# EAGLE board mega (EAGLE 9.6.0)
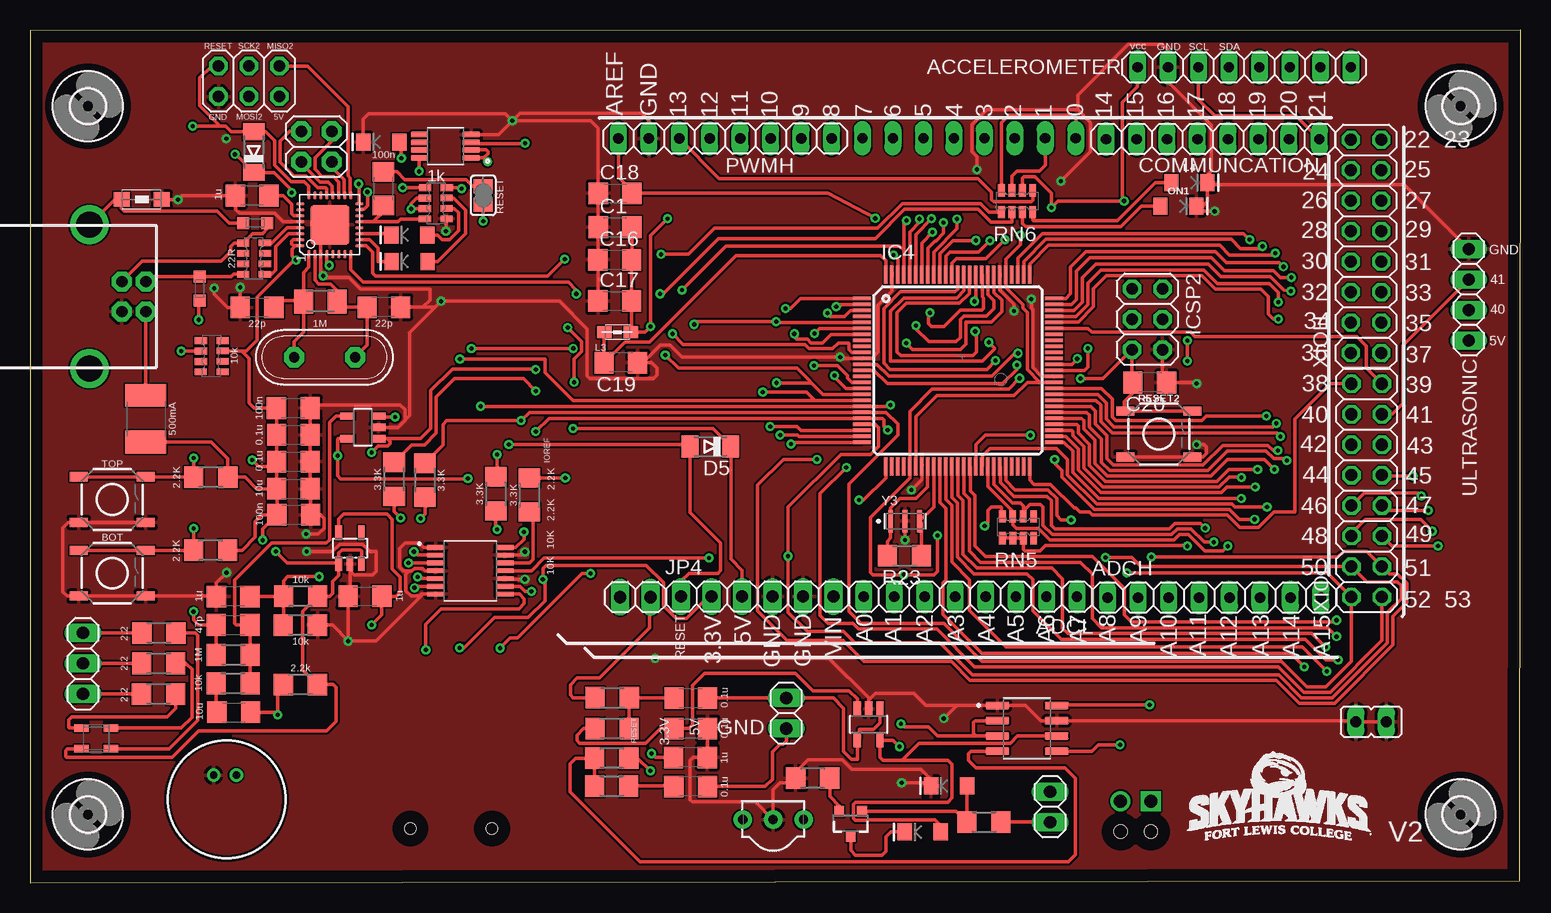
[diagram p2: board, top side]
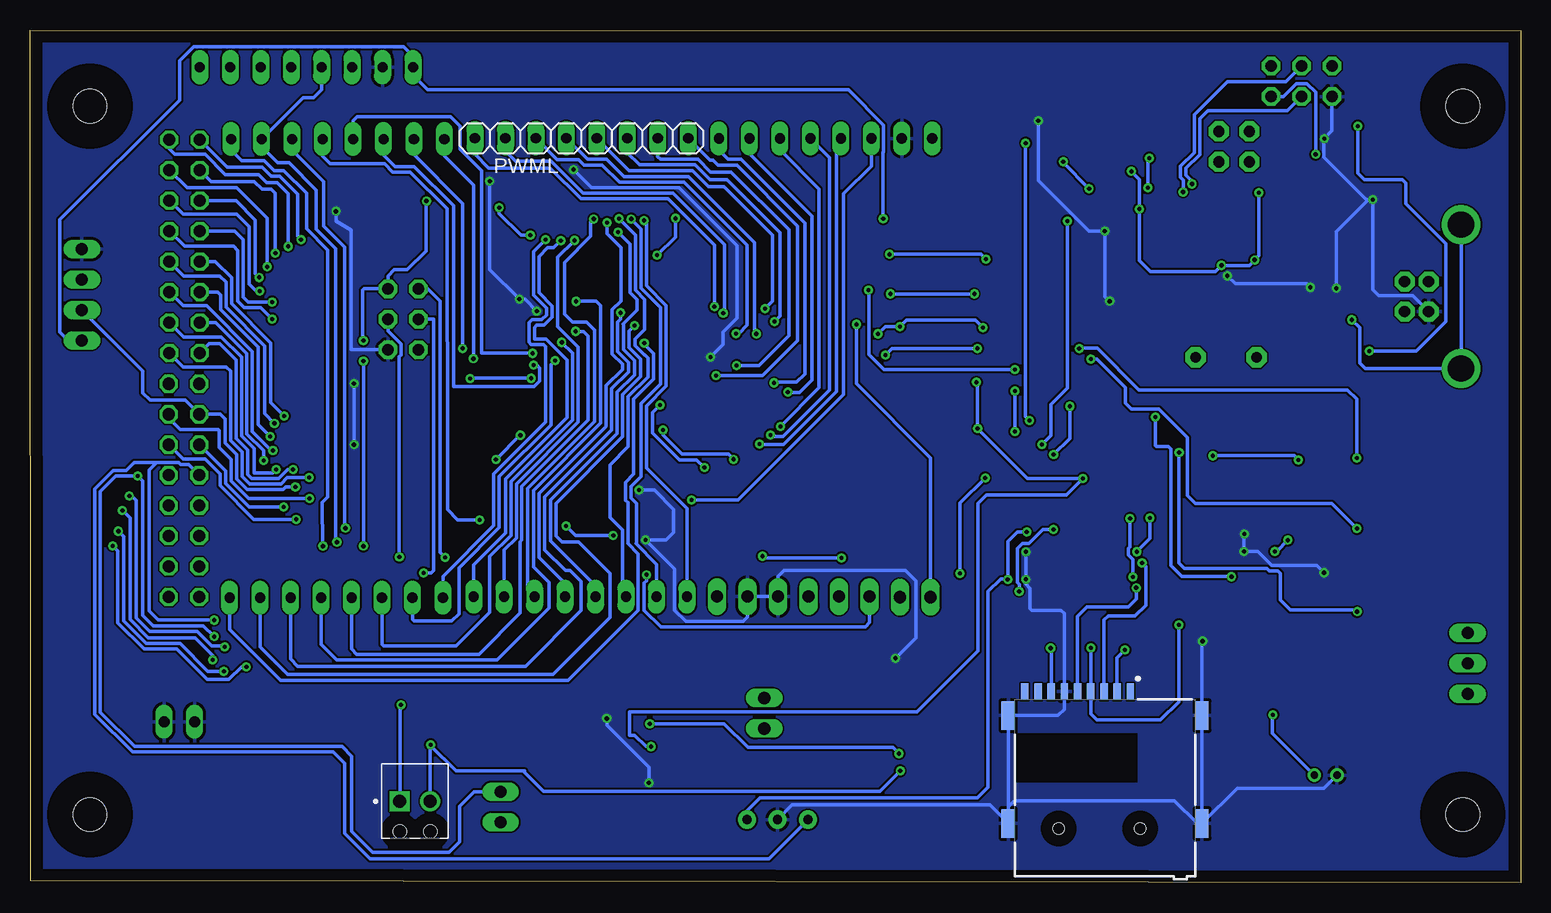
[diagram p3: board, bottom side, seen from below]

Size 124.26 x 71.1 mm. Coordinates in mm from the lower left corner, seen from the top.
Outline: 0,0 124.19,0.17 124.26,71.1 0.01,71.05 0,0
Copper layers (1*16): Top 0.035mm / dielectric 1.5mm / Bottom 0.035mm
Design rules "default": minimum track width 6mil, minimum drill 0.35mm, track to track 6mil, track to pad 6mil, pad to pad 6mil, via to via 6mil, smd to smd 6mil, copper to edge 40mil, drill to drill 6mil, minimum pad ring 10mil, minimum via ring 8mil, stop-mask expansion 4mil, vias tented up to drill 0mil, thermal gap 10mil
Net classes: 0 default: width 0.305 mm

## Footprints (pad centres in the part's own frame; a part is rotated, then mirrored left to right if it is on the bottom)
SMARTPRJ_1X08 = drill 0.85 pad 1.422 long: 1 -8.89,0; 2 -6.35,0; 3 -3.81,0; 4 -1.27,0; 5 1.27,0; 6 3.81,0; 7 6.35,0; 8 8.89,0
TACTILE_SWITCH_SMD_5.2MM = smd 1.524 x 0.762: 1 -2.794,1.905; 2 2.794,1.905; 3 -2.794,-1.905; 4 2.794,-1.905
SMARTPRJ_C1206 = smd 1.6 x 1.8: 1 -1.4,0; 2 1.4,0
LED-1206 = smd 1.2 x 1.4: A -1.5,0; C 1.5,0
DIODE_MINIMELF = smd 1.4 x 1.8: A 1.7,0; C -1.7,0
RCL_L1812 = smd 1.9 x 3.4: 1 -1.95,0; 2 1.95,0
2,8 = hole 2.8: 0,0
SOT23-5 = smd 0.6 x 1.2: 1 -0.95,-1.306; 2 0,-1.306; 3 0.95,-1.306; 4 0.95,1.306; 5 -0.95,1.306
INTEGRATEDCIRCUITS_TQFP100 = smd 1.5 x 0.3: 1 -8,6; 2 -8,5.5; 3 -8,5; 4 -8,4.5; 5 -8,4; 6 -8,3.5; 7 -8,3; 8 -8,2.5; 9 -8,2; 10 -8,1.5; 11 -8,1; 12 -8,0.5; 13 -8,0; 14 -8,-0.5; 15 -8,-1; 16 -8,-1.5; 17 -8,-2; 18 -8,-2.5; 19 -8,-3; 20 -8,-3.5; 21 -8,-4; 22 -8,-4.5; 23 -8,-5; 24 -8,-5.5; 25 -8,-6; 51 8,-6; 52 8,-5.5; 53 8,-5; 54 8,-4.5; 55 8,-4; 56 8,-3.5; 57 8,-3; 58 8,-2.5; 59 8,-2; 60 8,-1.5; 61 8,-1; 62 8,-0.5; 63 8,0; 64 8,0.5; 65 8,1; 66 8,1.5; 67 8,2; 68 8,2.5; 69 8,3; 70 8,3.5; 71 8,4; 72 8,4.5; 73 8,5; 74 8,5.5; 75 8,6 | smd 0.3 x 1.5: 26 -6,-8; 27 -5.5,-8; 28 -5,-8; 29 -4.5,-8; 30 -4,-8; 31 -3.5,-8; 32 -3,-8; 33 -2.5,-8; 34 -2,-8; 35 -1.5,-8; 36 -1,-8; 37 -0.5,-8; 38 0,-8; 39 0.5,-8; 40 1,-8; 41 1.5,-8; 42 2,-8; 43 2.5,-8; 44 3,-8; 45 3.5,-8; 46 4,-8; 47 4.5,-8; 48 5,-8; 49 5.5,-8; 50 6,-8; 76 6,8; 77 5.5,8; 78 5,8; 79 4.5,8; 80 4,8; 81 3.5,8; 82 3,8; 83 2.5,8; 84 2,8; 85 1.5,8; 86 1,8; 87 0.5,8; 88 0,8; 89 -0.5,8; 90 -1,8; 91 -1.5,8; 92 -2,8; 93 -2.5,8; 94 -3,8; 95 -3.5,8; 96 -4,8; 97 -4.5,8; 98 -5,8; 99 -5.5,8; 100 -6,8
2X03 = drill 0.95 pad 1.55 octagon: 1 -2.54,-1.27; 2 -2.54,1.27; 3 0,-1.27; 4 0,1.27; 5 2.54,-1.27; 6 2.54,1.27
SMARTPRJ_2X03 = drill 0.95 pad 1.55 octagon: 1 -2.54,-1.27; 2 -2.54,1.27; 3 0,-1.27; 4 0,1.27; 5 2.54,-1.27; 6 2.54,1.27
GCT_MEM2075-00-140-01-A = smd 0.62 x 1.4: P1 2.58,11.42; P2 1.48,11.42; P3 0.38,11.42; P4 -0.72,11.42; P5 -1.82,11.42; P6 -2.92,11.42; P7 -4.02,11.42; P8 -5.12,11.42; P9 -6.22,11.42 | smd 1.1 x 2.4: SH1 -7.6,0.42; SH2 -7.6,9.42; SH3 8.55,9.42; SH4 8.55,0.42 | hole 0.95: -3.4,0; 3.4,0
PHOENIX_1725656 = drill 1.1 square: 1 1.5,3.1 | drill 1.1: 2 4.04,3.1 | hole 1.1: 1.5,0.56; 4.04,0.56
SMARTPRJ_2X02 = drill 0.95 pad 1.676 octagon: 1 -1.27,-1.27; 2 -1.27,1.27; 3 1.27,-1.27; 4 1.27,1.27
1X03 = drill 1.016 long: 1 -2.54,0; 2 0,0; 3 2.54,0
1X06 = drill 1.016 long: 1 -6.35,0; 2 -3.81,0; 3 -1.27,0; 4 1.27,0; 5 3.81,0; 6 6.35,0
1X02 = drill 1.016 long: 1 -1.27,0; 2 1.27,0
JP1 = drill 0.914 long: 1 0,-1.27; 2 0,1.27
WUERTH-ELEKTRONIK_1206 = smd 1.35 x 1.2: 1 -1.7,0; 2 1.65,0
INDUTTANZE_0805 = smd 1.2 x 1: 1 -1.1,0; 2 1.1,0
SOT23-3 = smd 0.8 x 0.9: 1 -0.95,-1; 2 0.95,-1; 3 0,1.1
SMARTPRJ_M1206 = smd 1.6 x 2: 1 -1.4,0; 2 1.4,0
R1206 = smd 1.6 x 1.803: 1 -1.422,0; 2 1.422,0
SMARTPRJ_R1206 = smd 1.6 x 1.803: 1 -1.422,0; 2 1.422,0
JUMPER_SJ = smd 1.168 x 1.6: 1 -0.762,0; 2 0.762,0
RESISTOR-DIL_CAY16 = smd 0.559 x 1.016: 1 -1.283,-0.934; 2 -0.408,-0.94; 3 0.462,-0.943; 4 1.322,-0.942; 5 1.318,0.874; 6 0.452,0.877; 7 -0.42,0.877; 8 -1.289,0.883
TSOP382 = drill 0.762 pad 1.524: 1 -2.54,0; 2 0,0; 3 2.54,0
SMARTPRJ_SOT23-DBV = smd 0.55 x 1.2: 1 -0.95,-1.3; 2 0,-1.3; 3 0.95,-1.3; 4 0.95,1.3; 5 -0.95,1.3
SOP65P640X120-14N = smd 1.57 x 0.41: 1 -2.87,1.95; 2 -2.87,1.3; 3 -2.87,0.65; 4 -2.87,0; 5 -2.87,-0.65; 6 -2.87,-1.3; 7 -2.87,-1.95; 8 2.87,-1.95; 9 2.87,-1.3; 10 2.87,-0.65; 11 2.87,0; 12 2.87,0.65; 13 2.87,1.3; 14 2.87,1.95
SOP65P490X110-8N = smd 1.47 x 0.48: 1 -2.15,0.975; 2 -2.15,0.325; 3 -2.15,-0.325; 4 -2.15,-0.975; 5 2.15,-0.975; 6 2.15,-0.325; 7 2.15,0.325; 8 2.15,0.975
SMARTPRJ_MLF32 = smd 0.7 x 0.28: 1 -2.45,1.75; 2 -2.45,1.25; 3 -2.45,0.75; 4 -2.45,0.25; 5 -2.45,-0.25; 6 -2.45,-0.75; 7 -2.45,-1.25; 8 -2.45,-1.75; 17 2.45,-1.75; 18 2.45,-1.25; 19 2.45,-0.75; 20 2.45,-0.25; 21 2.45,0.25; 22 2.45,0.75; 23 2.45,1.25; 24 2.45,1.75 | smd 0.28 x 0.7: 9 -1.75,-2.45; 10 -1.25,-2.45; 11 -0.75,-2.45; 12 -0.25,-2.45; 13 0.25,-2.45; 14 0.75,-2.45; 15 1.25,-2.45; 16 1.75,-2.45; 25 1.75,2.45; 26 1.25,2.45; 27 0.75,2.45; 28 0.25,2.45; 29 -0.25,2.45; 30 -0.75,2.45; 31 -1.25,2.45; 32 -1.75,2.45 | smd 3.254 x 3.254: 33 0,0
WM-62PC/62PK = drill 0.6 pad 1: 1 -2.016,0.823; 2 -2.016,-1.077
GM1WA55311A = smd 1.2 x 0.65: 1 -1.535,0.856; 2 -1.535,-0.856; 3 0.9,-0.856; 4 0.9,0.856
MYSOIC8 = smd 1.97 x 0.6: 1 -2.47,1.905; 2 -2.47,0.635; 3 -2.47,-0.635; 4 -2.47,-1.905; 5 2.47,-1.905; 6 2.47,-0.635; 7 2.47,0.635; 8 2.47,1.905
1X04 = drill 1.016 long: 1 -3.81,0; 2 -1.27,0; 3 1.27,0; 4 3.81,0
SMARTPRJ_PN61729 = drill 0.95 pad 1.676 octagon: 1 1.25,4.71; 2 -1.25,4.71; 3 -1.25,2.71; 4 1.25,2.71 | drill 2.2: P$1 -6,0; P$2 6,0
2X08 = drill 1.016 octagon: 1 -8.89,-1.27; 2 -8.89,1.27; 3 -6.35,-1.27; 4 -6.35,1.27; 5 -3.81,-1.27; 6 -3.81,1.27; 7 -1.27,-1.27; 8 -1.27,1.27; 9 1.27,-1.27; 10 1.27,1.27; 11 3.81,-1.27; 12 3.81,1.27; 13 6.35,-1.27; 14 6.35,1.27; 15 8.89,-1.27; 16 8.89,1.27
SMARTPRJ_QS = drill 0.85 pad 1.676 octagon: 1 -2.54,0; 2 2.54,0
OSC_CSTNE16M0V530000R0 = smd 0.4 x 1.9: 1 -1.2,0; 2 0,0; 3 1.2,0
VARISTOR_CT/CN0603 = smd 1 x 1: 1 -1,0; 2 1,0

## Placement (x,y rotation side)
ACCELEROMETER  8x1  [SMARTPRJ_1X08]  101.22,68 180 top
ADCH  8x1  [SMARTPRJ_1X08]  98.73,23.78 0 top
ADCL  8x1  [SMARTPRJ_1X08]  78.39,23.85 180 top
BOT  MOMENTARY-SWITCH-SPST-SMD-5.2-REDUNDANT  [TACTILE_SWITCH_SMD_5.2MM]  6.85,25.81 0 top
C1  100n  [SMARTPRJ_C1206]  48.77,54.66 0 top
C2  100n  [SMARTPRJ_C1206]  21.98,30.67 180 top
C3  1u  [SMARTPRJ_C1206]  27.93,23.9 0 top
C5  100n  [SMARTPRJ_C1206]  29.46,57.88 90 top
C7  100n  [SMARTPRJ_C1206]  21.95,39.59 0 top
C8  1u  [SMARTPRJ_C1206]  18.52,57.29 180 top
C9  22p  [SMARTPRJ_C1206]  18.93,47.98 0 top
C11  22p  [SMARTPRJ_C1206]  29.49,47.99 180 top
C12  1u  [SMARTPRJ_C1206]  16.94,23.87 180 top
C13  47p  [SMARTPRJ_C1206]  16.93,21.5 0 top
C14  1u  [SMARTPRJ_C1206]  55.06,10.45 180 top
C15  0.1u  [SMARTPRJ_C1206]  55.07,8.03 180 top
C16  100n  [SMARTPRJ_C1206]  48.74,51.95 0 top
C17  100n  [SMARTPRJ_C1206]  48.74,48.52 0 top
C18  100n  [SMARTPRJ_C1206]  48.77,57.48 0 top
C19  100n  [SMARTPRJ_C1206]  49.25,43.36 180 top
C20  22p  [SMARTPRJ_C1206]  93.34,41.71 180 top
CC1  10u  [SMARTPRJ_C1206]  21.96,32.85 0 top
CC2  10u  [SMARTPRJ_C1206]  16.98,14.22 0 top
CC3  0.1u  [SMARTPRJ_C1206]  21.95,37.35 0 top
CC4  0.1u  [SMARTPRJ_C1206]  21.95,35.11 0 top
CC5  0.1u  [SMARTPRJ_C1206]  55.08,12.86 0 top
CC6  0.1u  [SMARTPRJ_C1206]  55.08,15.41 0 top
COMMUNCATION  8x1  [SMARTPRJ_1X08]  98.6,62 0 top
D1  INFRARED  [LED-1206]  74.41,4.24 180 top
D3  CD1206-S01575  [DIODE_MINIMELF]  18.65,60.93 90 top
D4  RED  [LED-1206]  76.61,8.08 180 top
D5  CD1206-S01575  [DIODE_MINIMELF]  56.72,36.38 180 top
F1  MF-MSMF050-2 500mA  [RCL_L1812]  9.65,38.7 270 top
H1  MOUNT-HOLE2.8  [2,8]  4.82,64.75 0 top
H2  MOUNT-HOLE2.8  [2,8]  119.25,64.75 0 top
H3  MOUNT-HOLE2.8  [2,8]  119.25,5.69 0 top
H4  MOUNT-HOLE2.8  [2,8]  4.82,5.69 0 top
IC2  OPA344N-SOT23  [SOT23-5]  27.75,37.98 90 top
IC3  OPA344N-SOT23  [SOT23-5]  69.91,13.21 180 top
IC4  ATMEGA2560-15AU  [INTEGRATEDCIRCUITS_TQFP100]  77.34,42.73 0 top
ICSP1  3x2 M  [2X03]  18.26,66.83 180 top
ICSP2  3X2 M  [SMARTPRJ_2X03]  93.14,46.99 270 top
J1  MEM2075_EE383  [GCT_MEM2075-00-140-01-A]  35.11,4.52 0 bottom
J2  1725656  [PHOENIX_1725656]  94.94,3.7 0 bottom
JP2  2x2 M-NM  [SMARTPRJ_2X02]  23.88,61.39 90 top
JP3  [1X03]  4.42,18.28 90 top
JP4  [1X06]  60.63,23.86 0 top
JP5  [1X02]  63.05,14.13 270 top
JP6  [1X02]  50.46,23.82 180 top
JP7  [JP1]  111.81,13.44 90 top
JP8  IR_TX  [1X02]  85.04,6.32 270 top
L  YELLOW  [LED-1206]  29.29,61.76 180 top
L1  BLM21  [WUERTH-ELEKTRONIK_1206]  9.28,56.98 180 top
L3  10uH  [INDUTTANZE_0805]  48.97,45.9 0 top
L4  YELLOW  [LED-1206]  96.65,58.37 0 top
ON1  GREEN  [LED-1206]  95.73,56.42 0 top
PWMH  8x1  [SMARTPRJ_1X08]  57.94,62.05 0 top
PWML  8x1  [SMARTPRJ_1X08]  78.28,62.08 180 bottom
Q1  600mA/40V  [SOT23-3]  68.4,4.97 180 top
R1  1M  [SMARTPRJ_M1206]  24.21,48.48 0 top
R3  10k  [R1206]  16.93,16.62 0 top
R4  2.2k  [R1206]  22.54,16.53 0 top
R5  10k  [R1206]  22.54,21.49 0 top
R6  10k  [R1206]  22.56,23.88 0 top
R7  2.2  [R1206]  10.71,15.73 0 top
R8  1M  [R1206]  16.94,19 180 top
R9  2.2  [R1206]  10.74,18.29 0 top
R10  2.2  [R1206]  10.75,20.81 0 top
R11  10k  [R1206]  48.48,8.08 180 top
R12  10k  [R1206]  48.49,10.39 0 top
R13  2.2K  [R1206]  48.53,15.44 180 top
R14  2.2K  [R1206]  48.52,12.86 0 top
R15  2.2K  [R1206]  15.07,33.82 0 top
R16  2.2K  [R1206]  15.06,27.73 0 top
R17  300  [R1206]  79.52,5.07 180 top
R18  2.2  [R1206]  65.25,8.72 0 top
R19  3.3K  [R1206]  30.35,33.63 90 top
R20  3.3K  [R1206]  32.92,33.56 90 top
R21  3.3K  [R1206]  38.82,32.43 90 top
R22  3.3K  [R1206]  41.63,32.34 90 top
R23  1M  [SMARTPRJ_R1206]  72.9,27.26 180 top
RESET2  MOMENTARY-SWITCH-SPST-SMD-5.2-REDUNDANT  [TACTILE_SWITCH_SMD_5.2MM]  94.11,37.42 0 top
RESET-EN  [JUMPER_SJ]  37.78,57.32 90 top
RN1  10k  [RESISTOR-DIL_CAY16]  15.12,43.89 90 top
RN2  1k  [RESISTOR-DIL_CAY16]  33.86,56.68 270 top
RN3  22R  [RESISTOR-DIL_CAY16]  18.65,52.02 90 top
RN5  10k  [RESISTOR-DIL_CAY16]  82.35,29.67 0 top
RN6  1k  [RESISTOR-DIL_CAY16]  82.27,56.85 0 top
RX  YELLOW  [LED-1206]  31.64,51.8 180 top
TOP  MOMENTARY-SWITCH-SPST-SMD-5.2-REDUNDANT  [TACTILE_SWITCH_SMD_5.2MM]  6.85,31.95 0 top
TX  YELLOW  [LED-1206]  31.62,54.01 180 top
U1  38kHz  [TSOP382]  61.95,5.27 0 top
U2  LP2985-33DBVR  [SMARTPRJ_SOT23-DBV]  26.68,27.9 0 top
U3  SN74LVC125APWR  [SOP65P640X120-14N]  36.7,26.01 0 top
U4  LMV358MM  [SOP65P490X110-8N]  34.63,61.42 180 top
U$1  SMARTPRJ_ATMEGA16U2-MU  [SMARTPRJ_MLF32]  25,54.86 90 top
U$2  PIC_MICROPHONE  [WM-62PC/62PK]  16.38,6.96 270 top
U$3  MY_RGB  [GM1WA55311A]  5.83,12.04 0 top
U$4  MYLM4862  [MYSOIC8]  83.12,12.88 0 top
ULTRASONIC  [1X04]  119.94,49.02 270 top
X2  USB-B_TH  [SMARTPRJ_PN61729]  4.95,48.87 270 top
XIOH  [2X08]  111.38,53.06 90 top
XIOL  [2X08]  111.43,32.72 90 top
Y1  16MHz  [SMARTPRJ_QS]  24.55,43.81 180 top
Y3  CSTNE16M0V530000R0  [OSC_CSTNE16M0V530000R0]  72.95,30.15 0 top
Z1  CG0603MLC-05E  [VARISTOR_CT/CN0603]  18.79,55.02 180 top
Z2  CG0603MLC-05E  [VARISTOR_CT/CN0603]  14.15,49.54 270 top

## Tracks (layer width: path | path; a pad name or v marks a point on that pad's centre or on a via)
8PB4
  Top 0.305: U$1.18 26.21,57.35 26.21,58.61 25.15,59.66 JP2.1
8PB5
  Top 0.305: U$1.19 25.75,58.42 25.29,58.88 24.37,58.88 23.76,59.5 23.76,60.44 25.15,61.84 JP2.3
8PB6
  Top 0.305: U$1.20 25.21,57.35 25.21,58.06 24.85,58.42 24.18,58.42 22.61,59.99 JP2.2
8PB7
  Top 0.305: U$1.21 24.75,57.87 24.66,57.97 23.99,57.97 23.03,58.93 22.01,58.93 20.85,60.08 20.85,61.85 21.66,62.66 JP2.4
+3V3  (via drill 0.35)
  Top 0.305: U2.5 25.73,30.34 26.14,30.75 29.76,30.75 30.21,30.3 30.21,26.15 30.85,25.51 30.85,24.24 30.5,23.9 C3.2 29.33,22.34 v28.49,21.5 | U3.14 40.48,27.95 41.17,28.64 v41.17,29.24 | JP4.2 56.55,23.86 54.73,22.04 53.84,22.04 52.8,23.08 52.8,25.02 51.35,26.47 43.04,26.47 42.77,26.2 42.77,25.32 v42.76,25.3 42.92,25.14 42.92,23.51 41.53,22.13 38.72,22.13 36.18,19.59 v35.82,19.59
  Bottom 0.305: v41.17,29.24 41.95,29.24 42.76,28.44 42.76,25.35 | 42.76,25.35 v42.76,25.3 | U1.3 64.49,6.02 63.42,7.09 45.29,7.09 44.4,7.98 44.4,24.29 43.33,25.35 42.76,25.35 | v28.49,21.5 28.49,15.1 30.02,13.57 35.3,13.57 35.83,14.09 J1.P4 35.83,19.58 v35.82,19.59
ADC0  (via drill 0.35)
  Top 0.305: R8.2 15.52,21.49 C13.1 14.03,21.5 13.63,21.9 v13.63,22.61 | v28.47,35.88 29,36.42 29.81,36.42 30.01,36.62 30.01,36.79 29.77,37.03 IC2.1 32.56,37.03 33.41,37.89 33.41,41.02 35.23,42.83 42.13,42.83 v42.16,42.8 | v54.35,49.41 58.04,53.09 72.49,53.09 72.84,52.74 IC4.97 72.84,54.99 v73.07,55.22
  Bottom 0.305: v13.63,22.61 13.78,22.76 19.22,22.76 20.05,23.59 20.05,25.81 20.22,25.98 20.93,25.98 21.17,26.22 28.02,26.22 28.48,26.69 28.48,35.87 v28.47,35.88 | v54.35,49.41 54.33,49.38 54.33,44.05 53.08,42.8 v42.16,42.8 | ADCL.8 69.5,31.19 72.87,34.56 72.87,39.75 71.22,41.4 71.22,48.14 72.87,49.79 72.87,55.02 v73.07,55.22
ADC1  (via drill 0.35)
  Top 0.305: v74.14,55.35 74.14,55.07 73.34,54.27 IC4.96
  Bottom 0.305: ADCL.7 72.04,26.56 73.76,28.28 73.71,28.32 73.71,31.63 74.16,32.08 74.16,33.04 73.33,33.87 73.33,34.78 | 73.33,34.78 73.33,39.94 71.68,41.59 71.68,47.95 73.33,49.6 73.33,54.51 74.14,55.32 v74.14,55.35 | 73.33,34.78
ADC2  (via drill 0.35)
  Top 0.305: v75.16,55.37 73.84,54.06 IC4.95
  Bottom 0.305: v75.16,55.37 73.79,54 73.79,49.41 73.01,48.63 73.01,46.14 73.81,45.34 73.81,44.78 73.02,44 73,44 72.74,43.74 72.74,42.18 74.4,40.53 74.4,36.37 75.92,34.85 75.92,30.45 74.88,29.42 74.88,24.15 ADCL.6
ADC3  (via drill 0.35)
  Top 0.305: v75.23,54.26 75.23,54.23 74.34,53.34 IC4.94
  Bottom 0.305: ADCL.5 77.12,24.75 80.88,28.5 80.88,31.91 75.31,37.48 75.31,40.91 73.87,42.35 73.87,43.53 74.79,44.45 74.79,46.55 74.81,46.57 73.66,47.73 73.66,48.63 74.24,49.22 74.24,53.27 v75.23,54.26
ADC4  (via drill 0.35)
  Top 0.305: IC4.93 74.84,52.9 75.45,53.51 75.5,53.51 76.15,54.16 v76.15,55.04
  Bottom 0.305: ADCL.4 79.66,24.97 81.81,27.12 81.81,32.48 76.5,37.79 76.27,38.01 76.22,38.06 76.22,41.46 74.88,42.8 74.88,43.25 75.73,44.1 75.73,47.79 75,48.52 75,52.96 76.15,54.1 v76.15,55.04
ADC5  (via drill 0.35)
  Top 0.305: v77.27,55.35 77.27,54.52 75.34,52.6 IC4.92
  Bottom 0.305: ADCL.3 82.78,24.44 82.78,32.86 77.62,38.03 77.21,38.44 77.21,46.1 77.85,46.74 79.02,46.74 79.7,47.42 79.7,51.72 77.52,53.9 77.52,55.1 v77.27,55.35
ADC6  (via drill 0.35)
  Top 0.305: IC4.91 75.84,52.45 76.92,53.53 78.83,53.53 v78.86,53.56
  Bottom 0.305: ADCL.2 84.74,27.74 83.72,28.76 83.72,33.25 78.56,38.41 78.56,44.68 80.26,46.38 80.26,52.15 v78.86,53.56
ADC7  (via drill 0.35)
  Top 0.305: v80.01,53.55 80.01,53.53 79.08,52.6 76.68,52.6 76.34,52.26 IC4.90
  Bottom 0.305: ADCL.1 87.28,26.52 84.63,29.17 84.63,33.68 79.5,38.81 79.5,43.59 81.25,45.34 82.19,45.34 82.19,46.31 82.01,46.49 81.42,46.49 80.75,47.16 80.75,48.1 81.84,49.19 81.84,52.2 81.1,52.94 80.62,52.94 v80.01,53.55
ADC8  (via drill 0.35)
  Top 0.305: IC4.89 76.84,51.65 77.24,52.05 79.7,52.05 v81.28,53.62
  Bottom 0.305: ADCH.1 89.84,25.56 85.6,29.8 85.6,34.1 81.28,38.42 81.28,44.71 81.46,44.88 82.47,44.88 82.65,45.06 82.65,46.71 82.42,46.94 81.61,46.94 81.21,47.34 81.21,47.91 82.29,49 82.29,52.61 v81.28,53.62
ADC9  (via drill 0.35)
  Top 0.305: IC4.88 77.34,49.51 77.11,49.28 72.57,49.28 71.17,47.88 71.17,43.34 71.7,42.8 79.75,42.8 v80.49,43.54
  Bottom 0.305: ADCH.2 92.38,21.97 92.23,21.82 89.1,21.82 88.49,22.43 88.49,26.25 85.14,29.61 85.14,33.86 80.82,38.18 80.82,43.21 v80.49,43.54
ADC10  (via drill 0.35)
  Top 0.305: IC4.87 77.84,49.35 77.26,48.77 72.84,48.77 71.72,47.65 71.72,43.49 79.4,43.49 80.41,44.5 80.41,44.58 v79.93,45.06
  Bottom 0.305: ADCH.3 94.92,19.89 94.77,19.74 88.75,19.74 85.95,22.53 85.95,27.2 84.17,28.98 84.17,33.44 79.05,38.57 79.05,44.15 79.93,45.04 v79.93,45.06
ADC11  (via drill 0.35)
  Top 0.305: IC4.86 78.3,50.68 78.3,49.14 77.47,48.31 73.07,48.31 72.29,47.53 72.29,44.25 72.59,43.94 78.6,43.94 78.92,44.26 78.92,45.98 v78.79,45.98
  Bottom 0.305: ADCH.4 97.46,19.48 97.03,19.05 86.84,19.05 83.41,22.48 83.41,28.42 83.26,28.57 83.26,33.04 77.72,38.58 77.72,45.59 78.1,45.98 v78.79,45.98
ADC12  (via drill 0.35)
  Top 0.305: v78.74,48.48 78.84,48.58 IC4.85
  Bottom 0.305: ADCH.5 100,19.89 98.7,18.6 85.31,18.6 81.01,22.9 81.01,25.05 82.29,26.34 82.29,32.71 76.68,38.32 76.68,48.11 77.05,48.48 v78.74,48.48
ADC13  (via drill 0.35)
  Top 0.305: v75.03,47.53 74.88,47.37 74.88,46.61 75.13,46.36 76.17,46.36 77.55,47.73 79.35,47.73 79.5,47.88 79.5,48.74 79.38,48.86 79.38,50.68 IC4.84
  Bottom 0.305: ADCH.6 102.54,18.67 101.93,18.06 82.95,18.06 78.31,22.71 78.31,25.12 79.22,26.04 79.63,26.04 81.35,27.77 81.35,32.16 75.77,37.75 75.77,41.2 74.37,42.6 74.37,43.39 75.27,44.29 75.27,46.76 75.03,47 v75.03,47.53
ADC14  (via drill 0.35)
  Top 0.305: v73.86,46.46 73.86,46.18 74.93,45.11 77.19,45.11 77.55,45.47 77.55,46.96 77.84,47.25 79.72,47.25 80.35,47.88 80.35,48.54 79.84,49.05 IC4.83
  Bottom 0.305: ADCH.7 105.08,19.66 102.79,17.38 80.67,17.38 75.92,22.13 75.92,25.78 78.54,28.4 79.91,28.4 80.42,28.91 80.42,31.62 74.85,37.19 74.85,40.72 73.35,42.22 73.35,43.67 74.33,44.64 74.33,45.99 v73.86,46.46
ADC15  (via drill 0.35)
  Top 0.305: v73.05,45.01 73.58,44.48 77.57,44.48 78,44.91 78,46.74 80.14,46.74 81,47.61 81,48.57 80.34,49.23 IC4.82
  Bottom 0.305: ADCH.8 107.62,21.11 103.38,16.87 79.41,16.87 73.56,22.72 73.56,27.44 74.42,28.29 74.42,31.69 74.62,31.89 74.62,33.38 73.94,34.06 73.94,40.34 72.29,41.99 72.29,44.12 73.05,44.88 v73.05,45.01
AREF  (via drill 0.35)
  Top 0.305: PWMH.1 49.05,58.83 50.17,57.71 C18.2 66.51,57.48 v70.46,55.4 | v71.98,52.33 72.34,51.97 IC4.98
  Bottom 0.305: v70.46,55.4 70.46,53.85 v71.98,52.33
BLUE
  Top 0.305: JP3.3 9.32,20.82 R10.1
D+
  Top 0.305: X2.3 9.37,51.83 15.95,51.83 16.74,52.61 16.74,53.06 17.02,53.34 RN3.5 18.57,54.14 19.38,54.14 19.79,54.54 Z1.1
D-
  Top 0.305: X2.2 10.08,50.54 Z2.1 16.78,50.54 16.97,50.73 RN3.8
DTR
  Top 0.305: RN2.4 30.92,55.35 30.67,55.11 28.6,55.11 | U$1.13 28.6,55.11 | 28.6,55.11 29.46,55.98 C5.1
GND  (via drill 0.35)
  Top 0.305: 26.53,23.89 C3.1 | 26.53,23.89 26.71,24.06 26.71,26.01 | 26.53,23.89 26.51,23.86 v26.51,20.14 26.53,20.17 | U3.1 32.82,27.96 32.45,28.34 31.28,28.34 30.8,27.86 30.8,26.32 31.14,25.99 31.6,25.99 | 31.6,25.99 31.32,25.71 31.32,24.35 31.75,23.91 32.48,23.91 32.62,24.06 U3.7 32.75,24.06 28.86,20.17 26.53,20.17 | U3.4 32.92,26.01 32.72,26.21 32.06,26.21 31.83,25.99 31.6,25.99 | U3.13 40.96,27.31 v41.25,27.6 | v41.25,25.31 39.63,25.31 U3.10 | U$1.33 24.25,54.11 U$1.3 24.25,50.8 v24.44,50.6 24.6,50.44 26.61,50.44 27.55,49.5 33.34,49.5 33.34,48.6 32.73,47.99 | 32.73,47.99 C11.1 | TOP.4 TOP.3 3.2,30.04 2.75,29.59 2.75,24.25 3.09,23.91 BOT.3 BOT.4 15.5,23.91 C12.2 15.54,25.01 v16.38,25.85 | R5.2 25.21,21.49 26.53,20.17 | v34.26,48.49 31.64,45.87 31.64,38.96 30.66,37.98 IC2.2 30.71,37.98 31.27,38.54 31.27,39.45 30.87,39.85 23.61,39.85 C7.2 CC3.2 CC4.2 CC1.2 23.38,32.82 C2.1 24.21,30.67 24.5,30.38 24.5,29.56 24.03,29.08 v23.03,29.08 | v15.36,49.57 15.36,49.08 16.47,47.98 C9.1 v17.53,49.64 | U2.2 26.71,26.57 26.71,26.01 | 26.71,26.01 27.04,25.68 28.57,25.68 28.85,25.96 28.85,27.62 28.34,27.62 27.73,28.23 25.82,28.23 25.21,27.62 v23.06,27.62 | JP7.1 JP7.2 110.46,13.51 U$4.7 84.25,13.51 82.98,14.78 U$4.1 77.26,14.78 | v34.67,54.32 34.67,55.29 RN2.5 | v34.26,48.49 33.76,47.99 32.73,47.99 | L.C 27.79,63.68 28.24,64.14 39.61,64.14 v40.21,63.54 | U4.4 39.06,62.39 v40.21,63.54 | v40.21,63.54 40.84,64.16 50.98,64.16 51.59,63.55 PWMH.2 | v40.21,63.54 46.73,63.54 47.37,62.9 C18.1 C1.1 47.37,51.97 C16.1 C17.1 | v34.26,48.49 44.15,48.49 46.46,46.18 46.46,42.27 46.68,42.04 51.99,42.04 52.27,42.32 52.27,42.9 51.81,43.36 C19.1 51.1,43.36 52.58,44.83 53.36,44.83 54.35,43.84 v67.54,43.84 67.65,43.73 IC4.11 70.17,43.73 70.7,44.25 70.7,48.18 71.84,49.33 IC4.99
  Top 0.305: ICSP2.6 94.41,42.04 C20.1 97.18,41.71 v97.26,41.63 | RESET2.3 RESET2.4 97.79,35.51 98.07,35.79 98.07,36.32 97.86,36.53 v97.26,36.53 | 98.15,58.22 L4.C 98.15,59.01 98.48,59.34 98.48,63.17 94.87,66.78 ACCELEROMETER.7 94.87,69.45 94.39,69.92 93.24,69.92 91.58,69.92 87.34,65.67 87.34,64.44 | 98.15,58.22 98.15,56.85 97.23,55.93 ON1.C 97.66,55.98 v98.75,55.98 | Y3.2 v72.95,28.58 | v73.48,32.74 74.34,33.6 IC4.32 | IC4.62 85.3,42.27 84.29,42.27 83.59,42.97 83.59,47.79 83.46,47.92 v83.46,48.67 | v82.02,47.68 82.02,48.24 80.84,49.41 IC4.81 | 87.34,64.44 79.77,64.44 78.54,63.21 78.54,60.95 78.93,60.55 v78.93,59.47 | 87.34,64.44 88.39,63.39 88.39,60.96 v85.93,58.5 | 77.26,14.78 74.68,14.78 73.68,15.78 70.46,15.78 69.91,15.23 IC3.2 69.92,14.52 69.92,15.41 66.61,18.72 v52.12,18.72 | CC5.2 56.48,10.47 C14.1 55.28,10.45 55.04,10.21 55.04,6.94 55.22,6.76 60.46,6.76 U1.2 61.95,7.75 62.53,8.33 63.44,8.33 R18.1 63.63,8.92 63.63,9.05 64.84,10.26 67.74,10.26 68.53,9.48 74.27,9.48 75.11,8.64 D4.C 74.86,8.33 v72.67,8.33 | v76.17,13.69 77.26,14.78 | ULTRASONIC.1 114.55,58.22 98.15,58.22 | L1.1 12.32,56.98 v12.33,56.97 12.66,57.29 C8.2 17.16,57.25 17.16,56.14 17.48,55.82 20.41,55.82 21.12,55.11 U$1.28
  Bottom 0.305: J1.SH1 J1.SH2 38.56,13.94 38.03,14.47 J1.P6 38.03,22.45 38.3,22.72 40.73,22.72 40.9,22.89 40.9,24.56 41.25,24.91 v41.25,25.31 v41.25,27.6 | J1.SH4 J1.SH3 26.56,20.09 v26.51,20.14 | J1.SH1 42.71,6.35 42.22,6.85 28.87,6.85 26.96,4.94 J1.SH4 | U$2.2 16.41,7.87 23.63,7.87 J1.SH4 | v15.36,49.57 15.36,54.3 12.69,56.97 v12.33,56.97 | v24.44,50.6 23.79,49.95 17.83,49.95 v17.53,49.64 | v16.38,25.85 16.97,26.44 20.75,26.44 21.92,27.62 v23.06,27.62 23.06,29.06 v23.03,29.08 | v34.26,48.49 34.67,48.89 v34.67,54.32 35.98,54.32 40.21,58.56 v40.21,63.54 | ICSP1.6 15.72,62.7 v16.37,62.05 16.4,62.01 16.4,60.5 12.87,56.97 v12.33,56.97 | v98.75,55.98 98.75,55.17 97.48,54.42 97.48,44.45 ICSP2.6 | v97.26,41.63 v97.26,36.53 | v73.48,32.74 72.21,32.74 70.61,31.14 70.61,29.19 71.22,28.58 v72.95,28.58 70.52,26.15 70.52,22.72 69.59,21.8 64.82,21.8 64.44,22.17 JP4.5 JP4.4 61.9,25.55 61.42,26.04 51.28,26.04 50.42,25.17 50.42,20.42 v52.12,18.72 | v82.02,47.68 83.01,48.67 v83.46,48.67 85.93,51.14 v85.93,58.5 | v67.54,43.84 66.5,44.88 66.5,45.93 65.33,47.09 65.3,47.09 65.3,53.11 70.15,57.97 77.43,57.97 v78.93,59.47 | v72.67,8.33 72.67,9.6 76.17,13.11 v76.17,13.69 | U1.2 60.74,6.48 44.25,6.48 J1.SH1 | X2.4 8.99,48.95 11.81,48.95 12.33,49.47 v12.33,56.97
  pour Top: 0,71.05 124.41,71.05 124.41,-0.1 0,-0.1
  pour Bottom: 0,71.05 0,-0.2 124.26,-0.2 124.26,71.05
GREEN
  Top 0.305: JP3.2 R9.1
L13  (via drill 0.35)
  Top 0.305: v35.97,57.87 35.88,57.96 RN2.8 | v38.13,60.11 37.8,60.44 U4.1 37.83,60.44 38.2,60.81 38.2,60.96 38.02,61.14 36.83,61.14 U4.2
  Bottom 0.305: v35.97,57.87 38.13,60.03 v38.13,60.11
M8RXD  (via drill 0.35)
  Top 0.305: U$1.9 28.02,53.11 28.55,52.58 28.55,50.83 28.8,50.57 43.15,50.57 v44.58,52 | v52.6,52.4 54.89,52.4 57.05,54.56 70.66,54.56 72.72,56.62 79.22,56.62 79.93,55.91 80.98,55.91 RN6.1
  Bottom 0.305: v44.58,52 44.98,52.4 v52.6,52.4
M8TXD  (via drill 0.35)
  Top 0.305: U$1.8 26.75,51.13 27.79,50.09 44.88,50.09 45.54,49.43 v45.54,49.1 | v52.53,49.1 52.78,49.1 57.41,53.73 70.47,53.73 72.91,56.16 79.03,56.16 80.09,55.1 81.84,55.1 81.86,55.12 RN6.2
  Bottom 0.305: v45.54,49.1 v52.53,49.1
MISO2
  Top 0.305: U$1.17 26.71,57.35 26.71,58.76 26.52,58.94 26.52,64.72 23.14,68.1 ICSP1.1
MISO_CARD  (via drill 0.35)
  Top 0.305: v39.18,19.56 40.03,20.41 40.66,20.41 46.03,25.79 v46.73,25.79 | v44.63,33.76 R22.2
  Bottom 0.305: v39.18,19.56 39.13,19.52 J1.P7 | v46.73,25.79 46.73,31.65 v44.63,33.76
MOSI2  (via drill 0.35)
  Top 0.305: U$1.16 27.45,58.21 v27.39,58.27
  Bottom 0.305: v27.39,58.27 27.39,58.5 27.89,59 27.89,59.57 26.75,60.7 26.75,63.69 26.09,64.36 19.46,64.36 ICSP1.4
MOSI_CARD  (via drill 0.35)
  Top 0.305: v31.55,26.67 U3.3
  Bottom 0.305: J1.P3 34.73,21.9 34.37,22.26 32.14,22.26 31.25,23.14 31.25,26.38 v31.55,26.67
N$1
  Top 0.305: R14.2 49.96,12.88 R13.1 49.99,15.41 CC6.1
N$2
  Top 0.305: RX.A 33.98,51.8 36.31,54.13 36.31,56.09 35.3,57.1 RN2.7
N$3  (via drill 0.35)
  Top 0.305: C12.1 21.12,23.87 R6.1 | R5.1 21.13,21.51 R6.1 | v30.45,38.83 29.15,38.83 IC2.3 | R6.1 21.13,25.17 21.49,25.52 v24.1,25.52
  Bottom 0.305: v30.45,38.83 v30.44,38.83 30.44,36.48 30.36,36.39 29.38,36.39 29.15,36.17 29.15,26.46 28.22,25.52 v24.1,25.52
N$4
  Top 0.305: TX.A 33.98,54.01 34.37,53.63 34.98,53.63 35.74,54.39 35.74,55.85 35.37,56.22 RN2.6
N$6
  Top 0.305: U$3.3 11.59,11.19 13.96,13.55 13.96,20.62 13.77,20.81 R10.2
N$7
  Top 0.305: R3.2 R8.1 18.36,21.47 C13.2 17.18,21.5 17.07,21.61 17.07,25.23 20.16,28.32 24.68,28.32 24.96,28.6 24.96,38.39 25.5,38.93 IC2.4
N$8  (via drill 0.35)
  Top 0.305: RN2.1 v31.08,57.96 | v30.96,60.42 30.96,61.59 L.A
  Bottom 0.305: v31.08,57.96 31.08,60.29 v30.96,60.42
N$9
  Top 0.305: ON1.A 92.66,56.42 90.93,54.69 83.01,54.69 82.73,54.97 RN6.3
N$10
  Top 0.305: R3.1 15.51,14.3 CC2.1
N$11  (via drill 0.35)
  Top 0.305: CC2.2 20.43,14.22 v20.64,14.01 20.64,16.05 R4.1
  Bottom 0.305: v20.64,14.01 20.69,13.97 20.69,12.46 U$2.1
N$12
  Top 0.305: U$3.4 12.6,12.9 13.5,13.8 13.5,17.78 12.99,18.29 R9.2
N$13
  Top 0.305: U$3.1 3.26,12.9 3.21,12.95 3.21,13.59 3.47,13.85 11.45,13.85 12.14,14.54 R7.2
N$14  (via drill 0.35)
  Top 0.305: U$4.2 78.81,13.51 78.66,13.36 78.66,12.45 78.87,12.24 U$4.3 75.64,12.24 74.9,12.98 72.87,12.98 v72.59,13.26 | v51.81,10.77 52.14,10.45 C14.2
  Bottom 0.305: v51.81,10.77 52.32,11.28 64.41,11.28 66.39,13.26 v72.59,13.26
N$15
  Top 0.305: U$4.4 78.46,10.97 78.23,10.75 78.23,10.21 78.87,9.58 86.28,9.58 87.15,8.72 87.15,2.31 86.56,1.73 50.85,1.73 45.01,7.57 45.01,9.93 45.46,10.39 R12.1 R11.2
N$16
  Top 0.305: R11.1 53.62,8.08 C15.2
N$17  (via drill 0.35)
  Top 0.305: v90.87,11.51 89.05,11.51 88.51,10.97 U$4.5 | R12.2 50.64,10.4 v51.71,9.32
  Bottom 0.305: J2.2 90.9,11.47 | 90.9,11.47 v90.87,11.51 | 90.9,11.47 88.75,9.32 83.03,9.32 83.03,9.22 81.43,7.62 53.41,7.62 v51.71,9.32
N$18  (via drill 0.35)
  Top 0.305: U$4.8 85.63,14.82 v93.34,14.82
  Bottom 0.305: J2.1 93.39,6.86 93.39,14.77 v93.34,14.82
N$19
  Top 0.305: JP6.1 51.66,23.75 51.66,21.24 47.5,17.07 45.62,17.07 45.06,16.51 45.06,15.65 45.27,15.44 R13.2
N$20
  Top 0.305: IC3.3 68.96,15.32 68.27,16 65.25,16 63.8,17.45 56.23,17.45 55.24,16.46 55.24,13.16 54.95,12.86 CC5.1 52.56,12.86 51.33,11.64 45.82,11.64 45.59,11.86 45.59,12.3 46.16,12.86 R14.1
N$21
  Top 0.305: IC3.1 70.86,13.33 70.33,12.8 69.14,12.8 69.14,12.08 IC3.4 68.96,10.29 68.48,10.29 67.82,10.95 67.82,14.56 66.98,15.4 JP5.1 CC6.2
N$24
  Top 0.305: L3.1 47.87,43.38 C19.2 49.58,45.1 50.8,45.1 51.64,45.1 58.85,52.3 70.92,52.3 71.34,51.88 IC4.100
N$26
  Top 0.305: RN6.4 83.59,55.25 83.64,55.2 90.65,55.2 93.83,58.37 L4.A
N$27
  Top 0.305: R17.1 85.02,5.07 JP8.2
N$28
  Top 0.305: Q1.1 77.21,5.97 R17.2 D4.A
N$29
  Top 0.305: Q1.2 67.45,6.41 66.67,7.19 R18.2
N$30
  Top 0.305: Q1.3 68.43,3.84 68.43,2.7 68.83,2.29 71.02,2.29 71.37,2.64 71.37,3.84 71.78,4.24 D1.C
N$33  (via drill 0.35)
  Top 0.305: U3.9 40.87,24.71 41.28,24.3 v41.8,24.3 | v38.93,29.46 38.82,29.57 R21.1
  Bottom 0.305: v41.8,24.3 41.8,24.89 41.93,25.02 41.93,27.88 41.53,28.28 40.99,28.28 40.62,28.66 40.28,28.99 39.81,29.46 v38.93,29.46
N$34  (via drill 0.35)
  Top 0.305: R20.1 32.92,30.75 v32.56,30.39 | U3.5 32.46,25.36 v32.32,25.51
  Bottom 0.305: v32.32,25.51 32.32,26.96 32.68,27.32 32.68,27.89 32.56,28.01 v32.56,30.39
N$35  (via drill 0.35)
  Top 0.305: U3.2 32.29,27.31 v32,27.61 | v30.9,30.42 30.35,30.96 R19.1
  Bottom 0.305: v32,27.61 30.9,28.71 v30.9,30.42
N$36
  Top 0.305: R22.1 41.94,30.61 41.94,26.97 41.63,26.66 U3.12
PA0  (via drill 0.35)
  Top 0.305: v101.67,53.62 101.16,54.13 84.38,54.13 82.34,52.09 IC4.78
  Bottom 0.305: XIOH.16 107.82,59.67 104.9,59.67 104.14,58.91 103.43,58.91 101.95,57.43 101.95,53.9 v101.67,53.62
PA1  (via drill 0.35)
  Top 0.305: v102.74,53.06 102.54,52.86 100.91,52.86 100.13,53.65 84.71,53.65 82.84,51.78 IC4.77
  Bottom 0.305: XIOH.15 112.65,61.19 112.19,60.73 109.68,60.73 108,59.06 105.21,59.06 104.52,58.37 103.66,58.37 102.74,57.46 v102.74,53.06
PA2  (via drill 0.35)
  Top 0.305: v103.81,52.5 103.66,52.35 100,52.35 99.19,53.17 84.91,53.17 83.34,51.6 IC4.76
  Bottom 0.305: XIOH.14 109.17,58.47 105.56,58.47 104.93,57.84 104.14,57.84 103.81,57.51 v103.81,52.5
PA3  (via drill 0.35)
  Top 0.305: v104.49,51.36 104.14,51.72 99.72,51.72 98.8,52.63 88.03,52.63 86.74,51.34 86.74,49.13 86.34,48.73 IC4.75
  Bottom 0.305: XIOH.13 111.17,57.94 107.03,57.94 104.49,55.4 v104.49,51.36
PA4  (via drill 0.35)
  Top 0.305: IC4.74 86.83,48.23 87.25,48.64 87.25,51.01 88.37,52.12 98.5,52.12 99.57,51.06 103.66,51.06 104.24,50.47 v105.15,50.47
  Bottom 0.305: XIOH.12 107.08,56.87 105.48,55.27 105.48,50.8 v105.15,50.47
PA5  (via drill 0.35)
  Top 0.305: v105.1,49.33 104.52,49.41 103.38,50.55 99.29,50.55 98.25,51.59 88.85,51.59 87.73,50.47 87.73,48.42 87.04,47.73 IC4.73
  Bottom 0.305: XIOH.11 111.5,55.73 107.03,55.73 105.99,54.69 105.99,49.91 105.41,49.33 v105.1,49.33
PA6  (via drill 0.35)
  Top 0.305: IC4.72 87.19,47.23 88.19,48.23 88.19,49.99 89.28,51.08 97.86,51.08 98.98,49.96 103.3,49.96 104.06,49.2 v104.06,48.42
  Bottom 0.305: XIOH.10 107.19,54.33 106.48,53.62 106.48,48.82 106.07,48.42 v104.06,48.42
PA7  (via drill 0.35)
  Top 0.305: IC4.71 85.38,46.77 87.38,46.77 88.64,48.04 88.64,49.53 89.74,50.63 97.68,50.63 98.79,49.51 102.61,49.51 103.25,48.87 103.25,47.4 103.66,46.99 v104.06,46.99
  Bottom 0.305: XIOH.9 111.38,53.06 107.29,53.06 106.95,52.72 106.95,48.5 106.4,47.96 105.03,47.96 v104.06,46.99
PB0  (via drill 0.35)
  Top 0.305: v38.93,35.7 38.93,33.95 R21.2 | v37.57,39.73 IC4.19 71.62,39.73 v71.73,39.83 | XIOL.1 112.7,20.2 108.38,15.88 106.18,15.88 104.05,18.01 78.74,18.01 75.59,21.16 69.07,21.16 68.62,21.62 66.52,21.62 65.86,22.28 65.86,32.44 v68.05,34.62
  Bottom 0.305: v38.93,35.7 37.57,37.06 v37.57,39.73 | v68.05,34.62 68.68,35.26 70.13,35.26 72.36,37.49 72.36,39.2 v71.73,39.83
PB1  (via drill 0.35)
  Top 0.305: R20.2 34.42,36.49 34.42,38.22 34.74,38.53 v40.94,38.53 41.63,39.23 IC4.20 71.37,39.23 72.34,38.26 72.34,37.33 68.25,33.24 68.25,22.63 69.26,21.62 76.2,21.62 79.35,18.47 104.27,18.47 104.29,18.49 106.45,16.34 108.02,16.34 110.16,18.47 XIOL.2 108.15,25.83 v91.44,25.83 | v41.27,61.67 41.23,61.64 36.89,61.64 U4.3
  Bottom 0.305: v40.94,38.53 41.27,38.86 v41.27,61.67 | ICSP2.3 90.6,46.99 90.6,26.04 90.8,25.83 v91.44,25.83
PB2  (via drill 0.35)
  Top 0.305: R19.2 31.81,36.51 32.89,36.51 33.87,37.49 33.87,40.51 35.4,42.04 39.4,42.04 39.41,42.03 41.13,42.03 v42.16,41 | v42.16,37.62 43.27,38.73 IC4.21 71.05,38.73 71.19,38.59 71.19,38.05 v71.5,37.75 | v93.47,27.16 109.04,27.16 109.52,27.64 111.43,27.64 XIOL.3 113.31,25.76 113.99,25.76 113.99,25.74 114.76,24.98 114.76,23.37 113.61,22.23 113.61,19.82 108.76,14.96 105.81,14.96 103.9,16.87 78.37,16.87 76.8,18.44 69.52,18.44 67.77,20.2 63.12,20.2 60.66,22.66 60.66,33.15 62.81,35.31 v65.61,35.31
  Bottom 0.305: v42.16,41 v42.16,37.62 | ICSP2.4 94.41,45.98 93.33,44.9 93.33,44.01 93.47,43.87 v93.47,27.16 | v65.61,35.31 66.04,35.74 69.92,35.74 71.5,37.32 v71.5,37.75
PB3  (via drill 0.35)
  Top 0.305: v89.66,27.13 91.84,27.13 92.61,26.37 XIOL.4 111.43,25.1 113.99,25.1 114.3,24.79 114.3,23.68 113.16,22.53 113.16,20.01 108.57,15.42 105.99,15.42 104.09,17.33 78.56,17.33 75.87,20.02 68.76,20.02 67.82,20.96 64.79,20.96 63.19,22.56 v63.19,27.23 63.19,31.32 67.59,35.72 70.08,35.72 70.74,36.38 70.74,37.98 70.49,38.23 IC4.22 | U3.11 41.81,26.01 42.87,27.08 v56.62,27.08
  Bottom 0.305: ICSP2.1 91.13,49.53 90.09,48.49 90.09,27.56 v89.66,27.13 | v56.62,27.08 63.04,27.08 v63.19,27.23
PB4  (via drill 0.35)
  Top 0.305: IC4.23 69.31,37.7 64.27,37.7 63.94,38.02 61.72,38.02 v61.7,38.04
  Bottom 0.305: v61.7,38.04 58.47,41.27 58.47,57.84 61.75,61.12 PWMH.6
PB5  (via drill 0.35)
  Top 0.305: v62.53,37.34 63.98,37.34 64.12,37.2 69.32,37.2 IC4.24
  Bottom 0.305: PWMH.5 57.61,60.45 57.61,41.1 61.49,37.21 62.41,37.21 v62.53,37.34
PB6  (via drill 0.35)
  Top 0.305: v63.45,36.58 63.59,36.73 IC4.25
  Bottom 0.305: PWMH.4 57.05,61.67 57.05,40.97 61.47,36.55 63.42,36.55 v63.45,36.58
PB7  (via drill 0.35)
  Top 0.305: PWMH.3 57.45,58.73 79.02,58.73 80.16,57.58 80.16,56.98 80.34,56.8 83.49,56.8 83.59,56.9 RN6.5 | IC4.26 71.34,33.75 69.49,31.91 v69.11,31.91
  Bottom 0.305: PWMH.3 54.13,59.77 56.44,57.46 56.44,40.72 65.25,31.91 v69.11,31.91
PC0  (via drill 0.35)
  Top 0.305: IC4.53 86.85,37.73 86.93,37.65 86.93,37.3 87.86,36.36 87.86,34.59 89.45,33 99.12,33 99.96,33.84 100.99,33.84 v100.99,33.79
  Bottom 0.305: XIOH.1 111.48,43.01 107.9,43.01 107.55,42.66 107.55,36.87 106.58,35.9 106.58,33.86 105.97,33.25 103.34,33.25 102.8,33.79 v100.99,33.79
PC1  (via drill 0.35)
  Top 0.305: v102.34,34.47 99.95,34.47 98.93,33.45 89.64,33.45 88.31,34.78 88.31,36.55 87.38,37.48 87.38,38.1 87.26,38.23 IC4.54
  Bottom 0.305: XIOH.2 109.32,44.96 108.46,44.96 107.09,43.6 107.09,37.06 106.12,36.09 106.12,34.05 105.78,33.71 103.53,33.71 102.77,34.47 v102.34,34.47
PC2  (via drill 0.35)
  Top 0.305: IC4.55 87.65,38.73 87.84,38.53 87.84,37.83 88.77,36.9 88.77,34.97 89.82,33.91 98.42,33.91 99.82,35.31 102.89,35.31 v103.73,34.47
  Bottom 0.305: XIOH.3 111.45,45.52 108.3,45.52 106.63,43.85 106.63,37.25 105.59,36.2 105.59,34.17 104.04,34.17 v103.73,34.47
PC3  (via drill 0.35)
  Top 0.305: IC4.56 88.06,39.23 88.3,38.99 88.3,38.02 89.33,36.99 89.33,35.05 90.01,34.37 98.19,34.37 99.82,35.99 103.03,35.99 103.67,35.36 104.62,35.36 v104.77,35.21
  Bottom 0.305: XIOH.4 108.77,46.71 106.18,44.12 106.18,37.44 104.77,36.03 v104.77,35.21
PC4  (via drill 0.35)
  Top 0.305: IC4.57 88.44,39.73 88.82,39.35 88.82,38.25 89.79,37.28 89.79,35.36 90.32,34.83 97.79,34.83 99.44,36.48 103.2,36.48 103.63,36.05 v104.01,36.05
  Bottom 0.305: XIOH.5 111.5,48.11 109.52,48.11 105.72,44.31 105.72,37.63 104.14,36.05 v104.01,36.05
PC5  (via drill 0.35)
  Top 0.305: IC4.58 88.87,40.23 89.28,39.82 89.28,38.46 90.23,37.51 103.94,37.51 v104.24,37.21
  Bottom 0.305: XIOH.6 108.63,49.25 108.38,49 108.38,47.8 105.23,44.65 105.23,38.2 v104.24,37.21
PC6  (via drill 0.35)
  Top 0.305: v103.88,38.31 103.6,38.02 90.37,38.02 89.74,38.65 89.74,40.01 89.02,40.73 IC4.59
  Bottom 0.305: XIOH.7 111.45,50.6 108.46,50.6 107.92,50.07 107.92,47.99 104.7,44.76 104.7,39.12 v103.88,38.31
PC7  (via drill 0.35)
  Top 0.305: IC4.60 89.33,41.23 90.24,40.31 90.24,38.81 90.53,38.53 97.68,38.53 98.07,38.92 v103.07,38.92
  Bottom 0.305: XIOH.8 108.81,51.79 107.47,50.45 107.47,48.28 104.19,45 104.19,40.03 v103.07,38.92
PD7
  Top 0.305: IC4.50 83.34,33.58 83.69,33.23 85.06,33.23 87.04,31.24 87.2,31.24 87.53,30.91 88.3,30.91 88.55,30.66 99.8,30.66 100.84,29.62 102.39,29.62 103.68,30.91 105.46,30.91 105.46,38.66 108.41,41.61 XIOL.16
PE0  (via drill 0.35)
  Top 0.305: RN6.8 80.98,63.38 81.58,63.99 86.94,63.99 87.17,63.76 PWML.8 | v67.21,48.04 67.39,48.23 IC4.2
  Bottom 0.305: PWML.8 87.17,60.73 86.03,59.59 80.9,59.59 78.33,57.03 71.07,57.03 67.21,53.17 v67.21,48.04
PE1  (via drill 0.35)
  Top 0.305: PWML.7 84.63,59.84 84.13,59.34 82.27,59.34 81.85,58.92 RN6.7 | v66.47,47.5 66.75,47.22 67.89,47.22 68.39,47.73 IC4.3
  Bottom 0.305: PWML.7 84.63,61.01 83.77,60.15 80.81,60.15 78.17,57.51 70.66,57.51 66.34,53.19 66.34,47.5 v66.47,47.5
PE3  (via drill 0.35)
  Top 0.305: IC4.5 62.26,46.73 v62.2,46.79 55.59,46.79 v55.37,46.56
  Bottom 0.305: v62.2,46.79 61.74,47.25 61.74,54.23 66.14,58.63 67.59,58.63 68.83,59.87 73.46,59.87 74.47,60.89 PWML.3 | JP6.2 49.19,35.43 55.37,41.61 v55.37,46.56
PE4  (via drill 0.35)
  Top 0.305: IC4.6 65.83,46.23 v65.4,45.8
  Bottom 0.305: PWML.6 80.31,60.3 78.51,60.3 78.05,59.85 76.55,59.85 75.13,58.42 69.75,58.42 64.49,53.17 64.49,46.48 65.17,45.8 v65.4,45.8
PE5  (via drill 0.35)
  Top 0.305: v63.71,45.77 63.71,45.55 63.92,45.34 64.79,45.34 65.12,45.01 66.07,45.01 66.78,45.73 IC4.7
  Bottom 0.305: PWML.5 77.8,60.33 76.2,60.33 74.75,58.88 69.37,58.88 63.85,53.37 63.85,45.92 v63.71,45.77
PG0  (via drill 0.35)
  Top 0.305: IC4.51 86.2,36.73 86.94,35.99 86.94,34.21 89.12,32.03 v100.96,32.03 | XIOL.13 113.56,39.07 114.45,39.96 114.45,44.81 ULTRASONIC.2
  Bottom 0.305: v100.96,32.03 106.04,32.03 107.49,33.48 107.49,35.28 108.48,36.27 108.48,37.7 108.56,37.77 111.73,37.77 112.7,38.74 XIOL.13
PG1  (via drill 0.35)
  Top 0.305: v102.13,33 99.77,33 99.31,32.54 89.26,32.54 87.4,34.4 87.4,36.17 86.35,37.23 IC4.52
  Bottom 0.305: v102.13,33 102.95,33 103.15,32.79 106.15,32.79 107.03,33.67 107.03,35.71 108.01,36.68 108.01,38.67 108.41,39.07 XIOL.14 111.33,40.24 114.25,40.24 114.86,40.85 114.86,42.67 ULTRASONIC.3
PG2
  Top 0.305: XIOL.15 111.38,42.93 111.38,44.76 110.59,45.55 97.1,45.55 96.75,45.9 88.52,45.9 88.19,46.23 IC4.70
PG5  (via drill 0.35)
  Top 0.305: IC4.1 64.23,48.73 63.39,47.88 v62.98,47.88
  Bottom 0.305: v62.98,47.88 62.35,48.52 62.35,54 66.39,58.04 67.69,58.04 69.04,59.39 74.32,59.39 PWML.4
PH3  (via drill 0.35)
  Top 0.305: IC4.15 68.51,41.73 68.15,42.09 68.15,42.29 67.31,43.13 v65.35,43.13
  Bottom 0.305: v65.35,43.13 63.5,43.13 61.01,45.62 61.01,54.46 65.81,59.26 67.51,59.26 68.58,60.33 71.7,60.33 71.93,60.56 PWML.2
PH4  (via drill 0.35)
  Top 0.305: v67.07,42.28 67.07,42.17 68.01,41.23 IC4.16
  Bottom 0.305: v67.07,42.28 63.21,42.28 60.26,45.23 60.26,54.75 65.33,59.82 66.9,59.82 67.33,60.25 67.56,60.25 PWML.1
PH5  (via drill 0.35)
  Top 0.305: TOP.1 TOP.2 13.62,33.85 R15.1 v13.65,35.41 | v45.29,44.55 45.28,44.55 v36.79,44.55 | v52.96,44 54.05,42.9 63.93,42.9 66.11,40.73 IC4.17 66.09,40.73 65.15,41.67 62.25,41.67 v62.23,41.68
  Bottom 0.305: v13.65,35.41 13.65,40.32 14.43,41.1 31.83,41.1 35.3,44.57 36.78,44.57 v36.79,44.55 | v45.29,44.55 52.4,44.55 v52.96,44 | v62.23,41.68 62.18,41.74 60.35,41.74 59.66,42.42 59.66,55.02 65,60.35 66.09,60.35 66.83,61.09 PWMH.8
PH6  (via drill 0.35)
  Top 0.305: BOT.1 BOT.2 9.65,27.73 R16.1 v13.63,29.53 v13.64,29.54 | v35.83,43.67 42.95,43.67 42.95,42.55 45.27,40.23 IC4.18 65.44,40.23 64.74,40.92 v61.09,40.92
  Bottom 0.305: v13.64,29.54 15.74,31.63 27.13,31.63 27.79,32.29 27.79,37.14 30.16,39.52 32.44,39.52 32.94,40.02 32.94,41.28 35.33,43.67 v35.83,43.67 | PWMH.7 64.29,60.81 59.05,55.58 59.05,41.91 60.09,40.87 61.03,40.87 v61.09,40.92
PL0  (via drill 0.35)
  Top 0.305: IC4.35 75.84,31.71 76.35,31.2 76.35,25.23 76.1,24.98 76.1,22.36 79.36,19.11 105.12,19.11 v106.22,18.01 | v117.37,28.1 113.51,28.1 XIOL.5
  Bottom 0.305: v106.22,18.01 106.63,18.01 107.69,16.94 109.5,16.94 112.04,19.48 114.75,19.48 116.94,21.67 116.94,27.66 v117.37,28.1
PL1  (via drill 0.35)
  Top 0.305: IC4.36 76.34,31.94 76.83,31.45 76.83,26.74 78.31,25.26 78.31,22.71 81.35,19.66 106.07,19.66 v108.1,17.63 | v116.89,29.31 115.92,30.28 111.33,30.28 110.16,29.11 XIOL.6
  Bottom 0.305: v108.1,17.63 109.45,17.63 111.76,19.94 114.56,19.94 116.46,21.84 116.46,28.88 v116.89,29.31
PL2  (via drill 0.35)
  Top 0.305: IC4.37 76.84,32.13 77.32,31.65 77.32,27.15 78.7,25.76 83.11,25.76 83.59,25.28 83.59,22.69 85.98,20.3 106.32,20.3 108.02,18.6 v109.04,18.6 | v116.56,31.04 113.1,31.04 XIOL.7
  Bottom 0.305: v109.04,18.6 109.04,18.98 110.49,20.42 114.4,20.42 115.92,21.95 115.92,30.43 116.53,31.04 v116.56,31.04
PL3  (via drill 0.35)
  Top 0.305: IC4.38 77.34,32.31 77.77,31.88 77.77,27.39 78.92,26.24 85.19,26.24 86.08,25.35 86.08,21.21 86.51,20.78 106.86,20.78 107.97,19.66 v108.02,19.66 | XIOL.8 111.23,32.51 115.72,32.51 v115.97,32.26
  Bottom 0.305: v108.02,19.66 108.13,19.76 109.12,19.76 109.6,20.24 | 109.6,20.24 | v115.97,32.26 115.8,32.26 115.42,31.88 115.42,22.09 114.28,20.96 110.31,20.96 109.6,20.24
PL4  (via drill 0.35)
  Top 0.305: IC4.39 77.84,32.47 78.31,32.01 78.31,27.65 79.23,26.72 87.55,26.72 88.54,25.73 88.54,22.02 89.3,21.26 108.18,21.26 v108.91,20.53 | v115.29,33.91 112.77,33.91 XIOL.9
  Bottom 0.305: v108.91,20.53 109.8,21.42 113.97,21.42 114.86,22.3 114.86,33.51 115.26,33.91 v115.29,33.91 117.12,33.91 118.39,32.64 118.39,14.23 115.52,11.36 98.25,11.36 97.43,10.54 97.43,4.3 95.68,2.54 89.33,2.54 88.44,3.43 88.44,6.38 87.23,7.59 JP8.1
PL5  (via drill 0.35)
  Top 0.305: IC4.40 78.38,34.68 78.38,32.68 78.79,32.28 78.79,28.07 79.65,27.21 88.56,27.21 91.24,24.53 91.24,22.33 91.79,21.77 108.79,21.77 v108.91,21.9
  Bottom 0.305: v108.91,21.9 113.56,21.9 114.32,22.66 114.32,34.42 113.69,35.05 | XIOL.10 111.05,34.88 111.69,34.88 111.87,35.05 113.69,35.05 | U1.1 62.67,2.01 95.91,2.01 98.04,4.14 98.04,9.96 98.98,10.9 115.71,10.9 118.85,14.04 118.85,32.83 117.31,34.37 116.25,34.37 115.57,35.05 113.69,35.05
PL6  (via drill 0.35)
  Top 0.305: v102.08,30.31 100.8,30.31 99.99,31.12 88.74,31.12 86.03,33.83 86.03,34.37 85.42,34.98 v85.42,35.28 | v83.39,37.32 79.63,37.32 78.84,36.53 IC4.41
  Bottom 0.305: v102.08,30.31 105.6,30.31 108.41,33.11 108.41,34.06 109.68,35.33 111.5,35.33 XIOL.11 | v85.42,35.28 v83.39,37.32
PL7  (via drill 0.35)
  Top 0.305: v103.12,31.32 100.43,31.32 100.18,31.58 88.93,31.58 86.49,34.02 86.49,35.31 85.57,36.22 80.01,36.22 79.38,35.6 79.38,34.77 IC4.42
  Bottom 0.305: XIOL.12 107.95,34.32 107.95,33.3 105.97,31.32 v103.12,31.32
PRE
  Top 0.305: C15.1 61.28,8.03 61.9,8.64 61.9,10.92 62.53,11.56 62.76,11.56 63.05,11.85 JP5.2
RD+
  Top 0.305: U$1.29 21.42,54.61 20.16,53.34 RN3.4
RD-
  Top 0.305: U$1.30 21.57,54.11 20.48,53.02 20.48,51.06 20.16,50.74 RN3.1
RED
  Top 0.305: JP3.1 9.28,15.74 R7.1
RESET  (via drill 0.35)
  Top 0.305: C5.2 30.6,59.28 31.25,58.64 36.33,58.64 36.89,58.08 RESET-EN.2 RESET-EN.1 v37.78,55.17 | v39.91,36.53 54.86,36.53 D5.A 55.02,30.89 57.58,28.32 57.58,26.04 57.35,25.81 54.94,25.81 54.28,25.15 JP4.1 | RESET2.2 RESET2.1 91.24,39.4 91.24,40.11 91.94,40.82 C20.2 91.84,41.81 91.84,44.43 ICSP2.5 89.46,42.04 v87.58,42.04 | v82.5,42.06 81.58,41.15 75.21,41.15 73.34,39.28 IC4.30 73.34,33.75 70.05,30.46 70.05,25.89 70.25,25.68 v72.87,25.68 75.36,25.68 75.64,25.96 v75.64,28.96 | RN5.8 80.98,30.55 80.98,31.27 80.93,31.32 80.16,31.32 79.87,31.03 79.87,30.04 v79.58,29.75
  Bottom 0.305: v39.91,36.53 39.15,37.3 39.15,39.87 37.78,41.24 v37.78,55.17 | v87.58,42.04 87.56,42.06 v82.5,42.06 | v79.58,29.75 78.79,28.96 v75.64,28.96 | JP4.1 54.28,21.69 54.63,21.34 71.67,21.34 73.06,22.72 73.06,24.98 72.87,25.17 v72.87,25.68
RESET2  (via drill 0.35)
  Top 0.305: U$1.24 23.25,58.06 22.84,58.47 21.77,58.47 20.39,59.84 20.39,61.88 19.64,62.63 D3.A 16.76,62.63 16.29,63.09 15.85,63.09 | RN1.6 v12.61,44.34 | 15.85,63.09 v13.57,63.09 | 15.85,63.09 14.15,64.79 14.15,67.11 15.14,68.1 ICSP1.5
  Bottom 0.305: v12.61,44.34 8.71,44.34 6.24,46.8 6.24,53.31 9.57,56.64 9.57,58.33 9.86,58.62 13.04,58.62 13.58,59.15 v13.58,63.08 v13.57,63.09
RXD1  (via drill 0.35)
  Top 0.305: IC4.45 80.88,34.68 80.88,33.35 82.03,32.21 84.78,32.21 85.14,31.85 85.14,29.8 85.44,29.49 94.97,29.49 95.45,29.97 97.56,29.97 v97.97,29.57
  Bottom 0.305: COMMUNCATION.6 102.41,61.06 99.8,58.45 99.8,54.74 98.04,52.99 98.04,29.64 v97.97,29.57
RXD2  (via drill 0.35)
  Top 0.305: v82.37,44.15 82.12,44.15 80.2,42.24 71.6,42.24 70.61,43.23 IC4.12
  Bottom 0.305: COMMUNCATION.4 97.33,63.55 97,63.88 89.2,63.88 88.42,63.1 88.42,61.18 86.61,59.37 86.61,44.15 v82.37,44.15
RXD3  (via drill 0.35)
  Top 0.305: v88.19,44.55 88.19,43.01 87.91,42.73 IC4.63
  Bottom 0.305: COMMUNCATION.2 92.25,60.71 88.19,56.64 v88.19,44.55
RXLED
  Top 0.305: U$1.10 28.33,53.61 29.01,52.93 29.01,51.8 RX.C
SCK2  (via drill 0.35)
  Top 0.305: U$1.15 27.49,56.15 27.85,56.15 28.13,56.44 v28.13,57.6
  Bottom 0.305: v28.13,57.6 28.13,58.6 28.35,58.81 28.35,59.76 27.21,60.89 27.21,64.03 24.45,66.79 19.57,66.79 ICSP1.3
SCK_CARD  (via drill 0.35)
  Top 0.305: v32.05,24.6 32.31,24.69 33.81,24.69 U3.6
  Bottom 0.305: J1.P5 36.93,22.22 36.14,23.02 32.68,23.02 32.05,23.65 v32.05,24.6
SCL  (via drill 0.35)
  Top 0.305: IC4.43 79.84,33.05 81.92,30.97 RN5.7 81.92,29.84 82.22,29.54 84.07,29.54 85.04,28.58 95.35,28.58 95.83,29.06 96.54,29.06 97.94,27.66 99.44,27.66 v99.85,28.07 | COMMUNCATION.8 105.54,63.96 98.75,63.96 97.41,65.31 ACCELEROMETER.6
  Bottom 0.305: COMMUNCATION.8 107.49,61.06 106.63,60.2 104.75,60.2 103.91,59.36 103.1,59.36 101.22,57.48 101.22,54.54 99.44,52.76 99.44,32.18 99.9,31.73 v99.85,28.07
SDA  (via drill 0.35)
  Top 0.305: IC4.44 80.34,33.2 81.89,31.65 82.56,31.65 82.8,31.41 RN5.6 82.8,31.01 83.34,31.55 84.22,31.55 84.45,31.32 84.45,29.81 85.23,29.04 95.16,29.04 95.64,29.52 96.76,29.52 97.88,28.4 v98.68,28.4
  Bottom 0.305: v98.68,28.4 98.78,28.5 98.78,52.89 100.4,54.51 100.4,57.76 102.67,60.02 103.61,60.02 104.95,61.37 COMMUNCATION.7 101.5,65.46 100.63,65.46 99.95,66.14 ACCELEROMETER.5
SS_CARD  (via drill 0.35)
  Top 0.305: v33,19.41 33,21.56 34.27,22.83 40.75,22.83 41.2,23.28 41.2,23.65 40.8,24.06 U3.8
  Bottom 0.305: J1.P2 33.66,15.97 33.66,18.75 v33,19.41
SUPPLY1_+5V  (via drill 0.35)
  Top 0.305: C1.2 50.17,51.97 C16.2 C17.2 50.14,45.97 L3.2 51.26,45.9 v51.74,46.38 51.74,53.98 v53.14,55.37 | RN6.6 82.72,58.75 82.85,58.88 83.77,58.88 85.14,57.51 v85.14,56.29 85.7,56.85 v91.21,56.85 91.06,57 91.06,65.1 92.33,66.37 ACCELEROMETER.8 | v96.47,45.21 v96.47,43.49 | v96.47,28.07 96.42,28.12 84.66,28.12 84.2,27.66 82.95,27.66 82.81,27.81 RN5.3 RN5.2 RN5.1 | v82.55,54 82.55,53.19 81.34,51.98 IC4.80 81.34,49.62 82.76,48.2 82.76,47.92 83.13,47.55 83.13,42.78 84.18,41.73 IC4.61 83.13,41.73 82.02,40.62 75.59,40.62 73.84,38.87 IC4.31 | v53.57,45.77 54.46,44.88 64.6,44.88 64.96,44.53 66.9,44.53 67.38,45.01 68.25,45.01 68.29,44.97 68.29,44.45 68.51,44.23 IC4.10 | JP4.3 59.36,26.06 58.42,27 D5.C 56.92,37.87 v45.26,37.87 | v45.36,41.74 45.36,43.66 45.97,44.27 45.97,45.14 v44.83,46.28 | RN2.2 32.22,57.08 31.77,56.63 v31.77,56.19 v31.77,56.18 31.8,56.21 RN2.3 | U$1.31 21.95,53.61 21.83,53.49 21.83,53.25 21.97,53.11 U$1.32 22.1,53.11 21.84,52.85 21.84,52.26 v22.17,51.93 22.03,51.93 18.92,48.83 18.92,45.25 18.02,44.35 17.65,44.35 | U$1.4 24.75,51.66 v24.93,51.48 | v21.82,57.53 21.82,57.77 20.36,59.23 D3.C 17.14,60.73 v17.09,60.73 | RN1.3 17.65,44.35 | 17.65,44.35 18.28,43.72 18.28,40 18.7,39.59 C7.1 CC3.1 CC4.1 | CC4.1 CC1.1 | CC1.1 20.58,32.82 C2.2 | CC1.1 18.9,32.85 17.93,33.82 R15.2 16.5,35.36 15.11,36.75 F1.2 | U$3.2 4.28,11.17 3.12,11.17 2.96,11.01 2.96,10.54 3.05,10.44 11.84,10.44 14.05,12.65 24.71,12.65 25.52,13.46 25.52,16.29 25.28,16.53 R4.2 22.74,17.75 22.74,22.64 R6.2 24.99,23.88 25.24,24.13 25.24,25.11 25.73,25.6 U2.1 | R16.2 17.68,27.73 18.78,28.82 18.78,30.13 19.33,30.67 C2.2
  Top 0.305: U2.3 27.63,27.67 27.54,27.77 26.01,27.77 25.73,27.49 U2.1 | U2.1 25.73,26.67 21.45,26.67 v20.49,27.62 | v19.4,28.57 19.4,29.49 C2.2 | IC2.5 25.7,37.03 25.63,36.95 25.63,35.62 v25.64,35.6 25.64,33.94 25.91,33.68 36.47,33.68 v36.5,33.71 | v18.52,35.26 19.06,34.72 20.16,34.72 CC4.1 | v32.45,59.32 32.45,60.41 U4.8 | U$4.6 82.32,12.24 81.71,11.64 74.12,11.64 72.67,10.19 | 72.67,10.19 71.12,10.19 70.86,10.45 IC3.5 70.87,11.89 71.96,11.89 v72.49,11.36 | 72.67,10.19 76.53,10.19 76.86,9.86 76.86,7.06 76.5,6.71 73.35,6.71 73.34,6.72 68.82,6.72 68.65,6.54 68.65,5.39 68.82,5.21 69.88,5.21 69.91,5.25 75.45,5.25 75.91,4.78 D1.A
  Bottom 0.305: v91.21,56.85 91.24,56.82 91.24,52.68 92.81,51.11 93.9,51.11 94.41,50.6 ICSP2.2 96.39,49.53 96.52,49.41 96.52,45.27 v96.47,45.21 | v96.47,43.49 v96.47,28.07 | v85.14,56.29 85.14,55.81 83.34,54 v82.55,54 | v53.57,45.77 52.96,46.38 v51.74,46.38 51.2,46.92 45.46,46.92 v44.83,46.28 | v45.36,41.74 45.26,41.63 v45.26,37.87 41.1,33.71 v36.5,33.71 37.87,32.34 44.52,32.34 45.24,31.63 45.24,19.33 50.32,14.25 74.29,14.25 74.29,12.3 73.86,12.3 72.92,11.36 v72.49,11.36 | ULTRASONIC.4 121.05,45.21 121.77,45.93 121.77,55.27 111.78,65.26 111.78,68.56 110.62,69.73 93.11,69.73 92.33,68.94 ACCELEROMETER.8 92.33,67.34 91.11,66.12 56.04,66.12 53.11,63.19 53.11,60.92 53.14,60.9 v53.14,55.37 | v21.82,57.53 21.82,52.28 v22.17,51.93 22.62,51.48 v24.93,51.48 25.44,50.97 30.87,50.97 31.77,51.87 v31.77,56.18 v31.77,56.19 31.77,58.62 32.45,59.29 v32.45,59.32 | v25.64,35.6 18.87,35.6 v18.52,35.26 | v19.4,28.57 20.34,27.62 v20.49,27.62 | v17.09,60.73 17.09,65.91 17.81,66.64 18.71,66.64 19.79,65.56 ICSP1.2
TP_VUCAP
  Top 0.305: C8.1 21.09,57.29 21.82,56.57 21.82,55.78 21.99,55.61 U$1.27
TXD1  (via drill 0.35)
  Top 0.305: IC4.46 81.34,33.54 82.12,32.77 84.87,32.77 85.6,32.04 85.6,30.61 85.95,30.25 v86.79,30.25
  Bottom 0.305: COMMUNCATION.5 99.87,60.58 99.24,59.95 94.7,59.95 94.02,59.26 92.56,59.26 89.48,56.19 89.46,34 89.46,31.12 88.59,30.25 v86.79,30.25
TXD2  (via drill 0.35)
  Top 0.305: v82.27,43.16 82.27,42.8 81.08,41.61 71.48,41.61 70.36,42.73 IC4.13
  Bottom 0.305: COMMUNCATION.3 94.79,60.68 93.83,59.72 92.23,59.72 88.95,56.44 88.95,41.35 82.24,41.35 81.76,41.83 81.76,42.93 81.99,43.16 v82.27,43.16
TXD3  (via drill 0.35)
  Top 0.305: v87.3,43.69 86.83,43.23 IC4.64
  Bottom 0.305: COMMUNCATION.1 89.71,60.58 87.3,58.17 v87.3,43.69
TXLED
  Top 0.305: TX.C 29.79,54.01 29.69,54.11 U$1.11
UNSHIELD  (via drill 0.35)
  Top 0.305: X2.P$1 7.06,56.98 7.6,56.98 | 7.6,56.98 L1.2 | Z1.2 16.59,55.02 15.59,56.01 7.84,56.01 7.6,56.25 7.6,56.98 | v14.07,46.94 14.07,48.46 Z2.2
  Bottom 0.305: X2.P$1 X2.P$2 12.96,42.87 13.41,43.33 13.41,46.28 v14.07,46.94
XT1
  Top 0.305: U$1.1 23.25,51.32 22.8,50.87 22.8,48.86 22.81,48.85 R1.1 | Y1.2 22.01,45.13 22.81,45.93 R1.1 | R1.1 22.81,48.56 20.91,48.56 C9.2
XT2
  Top 0.305: U$1.2 23.76,50.23 24.07,49.92 25.08,49.92 25.61,49.39 R1.2 26.1,47.99 C11.2 28.09,44.81 Y1.1
XTAL1
  Top 0.305: R23.1 74.32,29.98 Y3.3 75.34,31.35 IC4.34
XTAL2
  Top 0.305: R23.2 71.47,28.48 71.75,28.75 Y3.1 71.75,31.26 72.52,32.03 73.84,32.03 74.82,33.01 74.82,34.7 IC4.33
XUSB
  Top 0.305: X2.1 9.66,40.65 F1.1

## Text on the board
tPlace: RESET | SCK2 | MISO2 | vcc | GND | SCL | SDA | GND | MOSI2 | 5V | AREF | GND | 13 | 12 | 11 | 10 | 9 | 8 | 7 | 6 | 5 | 4 | 3 | 2 | 1 | 0 | 14 | 15 | 16 | 17 | 18 | 19 | 20 | 21 | 100n | 22 23 | 1k | 24 | 25 | 1u | RESET | 26 | 27 | 28 | 29 | GND | 22R | 30 | 31 | 41 | 32 | 33 | 40 | 22p | 1M | 22p | 34 | 35 | 5V | 10k | 36 | 37 | 38 | 39 | 100n | 500mA | 40 | 41 | 0.1u | IOREF | 42 | 43 | TOP | 0.1u | 2.2K | 3.3K | 3.3K | 2.2K | 10u | 3.3K | 44 | 45 | 3.3K | 100n | 2.2K | 46 | 47 | BOT | 10K | 49 | 2.2K | 48 | 10K | 50 | 51 | 10k | 1u | 1u | 52 53 | 47p | 2.2 | 10k | 5V | A0 | A1 | A2 | A3 | A4 | A5 | A6 | A7 | A8 | A9 | 1M | RESET | VIN | A10 | A11 | A12 | A13 | A14 | A15 | 2.2 | 2.2k | 3.3V | GND | GND | 10k | 2.2 | 0.1u | 10u | RESET | 3.3V | 5V | GND | 0.1u | 1u | 0.1u | V2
